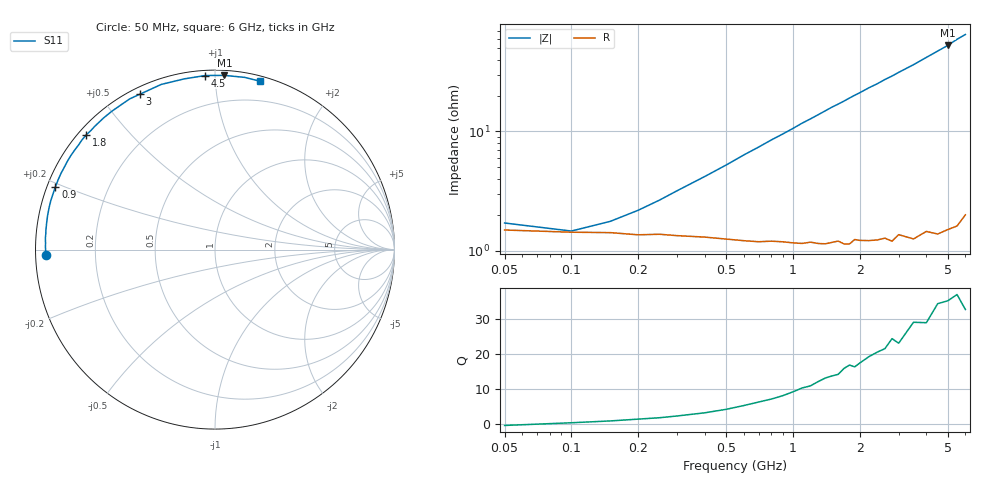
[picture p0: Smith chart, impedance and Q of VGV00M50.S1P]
! Infineon Technologies  Discrete & RF Semiconductors
! BB 831
! Si Tuning Diode in SOD323
! VR =
! S-Parameters:  July  1999
# GHz  S  MA  R  50
!  f  S11
! GHz  MAG  ANG
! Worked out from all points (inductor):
!   34 points, 50 MHz to 6 GHz, reference 50 ohm
!   read as one part to ground: L = 1.63 nH near 400 MHz
!   highest Q = 35.2 at 5 GHz (marker M1), where L = 1.68 nH
!   S11 on the Smith chart (normalised r, x): 50 MHz: 0.03, -0.02; 900 MHz: 0.02, +0.19; 1.8 GHz: 0.02, +0.38; 3 GHz: 0.03, +0.63; 4.5 GHz: 0.03, +0.95; 6 GHz: 0.04, +1.30
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0.05  0.9423 -178.1
0.1  0.9446 179.3
0.15  0.9451 177.6
0.2  0.9473 176.1
0.3  0.9482 173.4
0.5  0.9518 168.4
0.6  0.9535 165.8
0.7  0.9546 163.4
0.8  0.9545 160.9
0.9  0.9553 158.6
1.1  0.9574 153.7
1.4  0.959 146.9
1.5  0.9584 144.6
1.6  0.9578 142.6
1.7  0.9606 140.5
1.8  0.9611 138.3
1.9  0.9583 136.2
2.2  0.9609 130.2
2.4  0.9616 126.7
2.6  0.9616 122.8
2.8  0.9649 119.5
3  0.9617 115.9
3.5  0.9678 108.0
4  0.9665 100.2
4.5  0.9714 93.2
5  0.972 86.9
5.5  0.9737 80.2
6  0.9709 75.0
